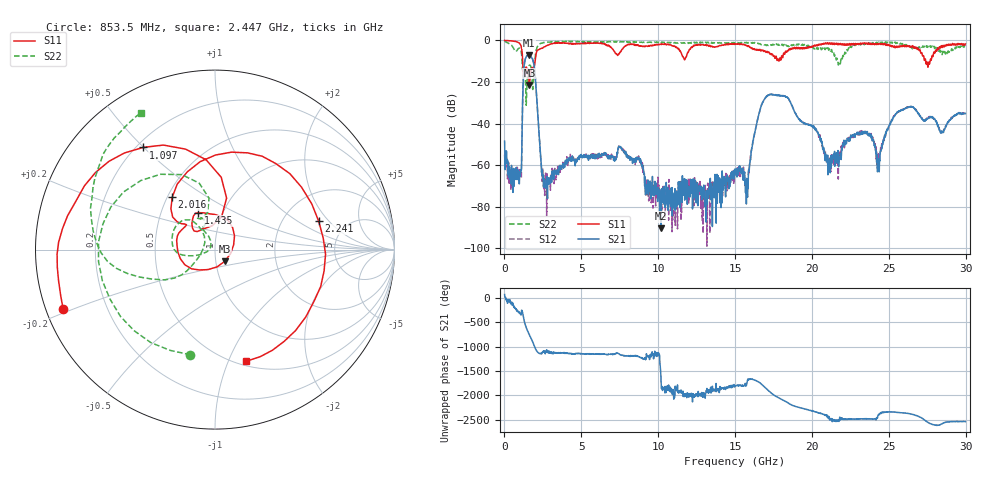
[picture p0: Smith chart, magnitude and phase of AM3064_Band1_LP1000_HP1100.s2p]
# Hz S DB R 50.0
!freq dBS11 angS11 dBS21 angS21 dBS12 angS12 dBS22 angS22
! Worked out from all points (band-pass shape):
!   1600 points, 10 MHz to 29.98 GHz, reference 50 ohm
!   highest |S21| = -7.04 dB at 1.584 GHz (marker M1); lowest = -90.4 dB at 10.19 GHz (marker M2)
!   |S21| within 3 dB of the highest: 1.322 GHz to 1.872 GHz (550.1 MHz wide, 34.4 % of centre)
!   lowest |S11| = -21.4 dB at 1.622 GHz (marker M3), VSWR 1.19, Z = 55.4 - j7.21 ohm
!   |S11| at or under -10 dB: 1.187 GHz to 1.988 GHz (801.2 MHz wide, 50.5 % of centre); 27.4 GHz to 27.68 GHz (283.6 MHz wide, 1.03 % of centre)
!   |S22| runs from -31.2 to -0.4 dB; largest |S21 - S12| = 0.0065
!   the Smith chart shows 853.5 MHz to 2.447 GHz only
!   S11 on the Smith chart (normalised r, x): 853.5 MHz: 0.05, -0.19; 1.097 GHz: 0.23, +0.50; 1.435 GHz: 0.77, +0.33; 2.016 GHz: 0.53, +0.36; 2.241 GHz: 3.15, +1.56; 2.447 GHz: 0.55, -1.16
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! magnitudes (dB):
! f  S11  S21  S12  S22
! 10 MHz  0.0  -48.5  -55.0  -0.4
! 853.5 MHz  -0.8  -63.5  -61.0  -4.4
! 1.097 GHz  -3.1  -62.5  -66.4  -5.7
! 1.435 GHz  -12.9  -7.7  -7.6  -27.2
! 1.584 GHz  -19.4  -7.0  -7.1  -12.2
! 1.622 GHz  -21.4  -7.1  -7.1  -12.0
! 2.016 GHz  -8.5  -18.8  -18.7  -7.0
! 2.241 GHz  -4.5  -43.9  -43.4  -2.0
! 2.447 GHz  -3.8  -64.8  -67.8  -1.3
! 5.015 GHz  -1.4  -56.1  -55.9  -0.8
! 7.545 GHz  -5.6  -51.2  -51.5  -0.7
! 10 GHz  -2.0  -73.2  -70.6  -0.9
! 10.19 GHz  -1.9  -90.4  -72.0  -1.0
! 15 GHz  -1.9  -62.1  -63.1  -1.4
! 15.77 GHz  -2.5  -68.7  -68.9  -1.1
! 17.16 GHz  -5.6  -26.3  -26.2  -2.5
! 19.99 GHz  -3.3  -41.2  -40.8  -3.1
! 21.12 GHz  -1.3  -58.5  -56.1  -4.6
! 23.44 GHz  -1.4  -44.2  -44.1  -1.5
! 24.34 GHz  -1.9  -57.0  -56.7  -1.1
! 25 GHz  -2.0  -41.3  -42.1  -1.1
! 29.98 GHz  -1.7  -35.1  -35.4  -3.2
